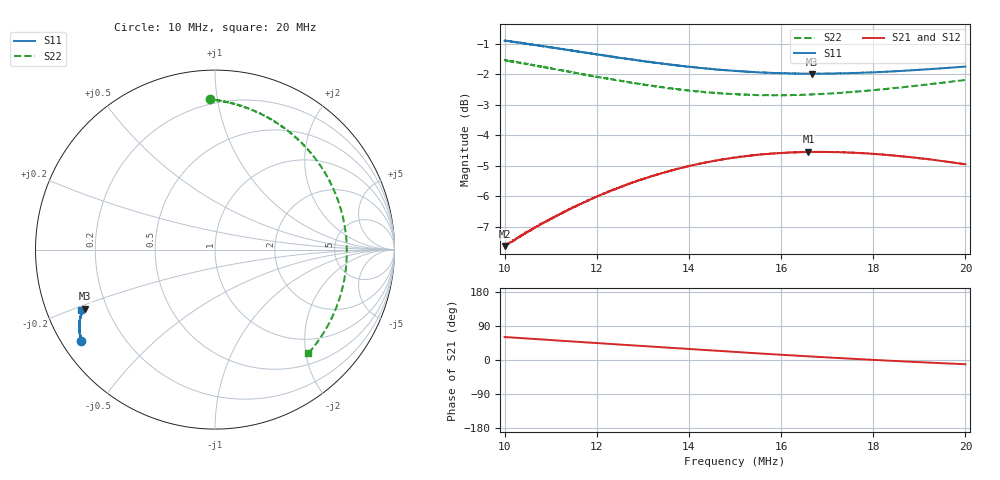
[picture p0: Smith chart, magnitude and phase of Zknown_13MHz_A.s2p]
!Agilent Technologies,N5242A,MY49421279,A.09.90.21
!Agilent N5242A: A.09.90.21
!Date: Monday, January 30, 2023
!Caliblation kit: 85033D 3.5mm Calibration Kit
!DUT Connector Gender Port1: male
!DUT Connector Gender Port2: female
!S2P File: Measurements: S11, S21, S12, S22:
# Hz S  dB  R 50
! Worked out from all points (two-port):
!   2001 points, 10 MHz to 20 MHz, reference 50 ohm
!   highest |S21| = -4.53 dB at 16.59 MHz (marker M1); lowest = -7.6 dB at 10.01 MHz (marker M2)
!   |S21| within 3 dB of the highest: 10.08347 MHz to 10.08822 MHz (4.753 kHz wide, 0.0471 % of centre); 10.1 MHz to end of sweep
!   lowest |S11| = -2.0 dB at 16.67 MHz (marker M3), VSWR 8.77, Z = 5.96 - j10.7 ohm
!   |S11| at or under -10 dB: nowhere
!   |S22| runs from -2.7 to -1.5 dB; largest |S21 - S12| = 0.0029
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1e7  -0.91 -145.7  -7.61 60.5  -7.64 60.7  -1.54 92.0
1.0005e7  -0.91 -145.7  -7.63 60.6  -7.64 60.6  -1.53 91.9
1.038e7  -0.98 -147.2  -7.27 57.5  -7.29 57.7  -1.63 87.1
1.088e7  -1.09 -148.9  -6.83 53.6  -6.84 53.8  -1.78 80.6
1.126e7  -1.18 -150.0  -6.51 50.6  -6.54 50.8  -1.88 75.4
1.167e7  -1.27 -151.1  -6.23 47.3  -6.24 47.5  -2.00 69.6
1.21e7  -1.37 -152.0  -5.94 43.9  -5.96 44.1  -2.11 63.4
1.247e7  -1.46 -152.7  -5.73 41.0  -5.73 41.1  -2.21 58.0
1.2945e7  -1.56 -153.6  -5.45 37.2  -5.46 37.3  -2.31 50.8
1.3335e7  -1.64 -154.1  -5.27 34.1  -5.27 34.2  -2.40 44.9
1.3825e7  -1.73 -154.7  -5.07 30.3  -5.08 30.3  -2.50 37.2
1.4185e7  -1.78 -154.9  -4.95 27.4  -4.95 27.6  -2.55 31.6
1.465e7  -1.85 -155.2  -4.81 23.9  -4.82 24.0  -2.62 24.3
1.5e7  -1.89 -155.4  -4.73 21.2  -4.73 21.3  -2.66 18.8
1.5735e7  -1.95 -155.5  -4.61 15.8  -4.61 15.8  -2.69 7.6
1.617e7  -1.97 -155.6  -4.56 12.7  -4.57 12.7  -2.69 1.0
1.6595e7  -1.99 -155.6  -4.53 9.7  -4.55 9.7  -2.67 -5.2
1.667e7  -1.99 -155.6  -4.54 9.1  -4.55 9.2  -2.66 -6.3
1.744e7  -1.97 -155.5  -4.56 3.9  -4.56 4.0  -2.60 -17.1
1.8335e7  -1.91 -155.5  -4.65 -1.7  -4.65 -1.6  -2.48 -28.9
1.921e7  -1.84 -155.6  -4.78 -6.9  -4.79 -6.8  -2.33 -39.4
2e7  -1.75 -155.7  -4.95 -11.2  -4.96 -11.1  -2.19 -48.0
